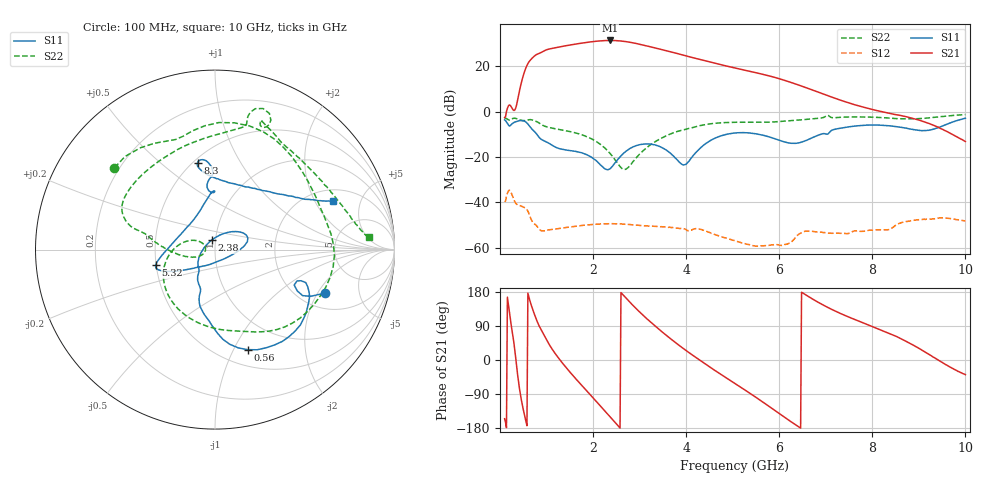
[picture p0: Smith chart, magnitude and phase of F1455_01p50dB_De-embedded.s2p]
! Integrated Device Technology
! Corporate Headquarters
! 6024 Silver Creek Valley Road
! San Jose, CA 95138  USA
! Phone:  1-408-284-8200
! Toll Free:  1-800-223-1366
! Webpage:  http://www.idt.com/
! Timing and RF Division
! 515 Groton Road, Suite 102
! Westford, MA 01886-6024
! Device:  F1455
! Description: 6-bit 0.5 dB Transmit Variable Gain Amplifier
! Frequency:  1400.0 -  2300.00 MHz
! Package:  6x6 mm Thin QFN Plastic Package: 28 pin
! State:  3
! Atten State:  1.5 dB
! Voltage:  +5.00 Volts
! Current:  214.186 mA
! Data:  The device was measured on a the F1455 evaluation board which has
!  individual transmission lines to the RF pins.  Data was collected
!  using a calibrated network analyzer.  The evaluation board was
!  de-embedded using a TRL calibration technique.
!  The reference plane is the edge of the package pin.
!  Pin  1 = CSb
!  Pin  2 = DATA
!  Pin  3 = CLK
!  Pin  4 = RSET
!  Pin  5 = GND
!  Pin  6 = RFIN  = Port 1
!  Pin  7 = GND
!  Pin  8 = NC
!  Pin  9 = NC
!  Pin 10 = NC
!  Pin 11 = NC
!  Pin 12 = NC
!  Pin 13 = NC
!  Pin 14 = /STBY
!  Pin 15 = GND
!  Pin 16 = RFOUT  = Port 2
!  Pin 17 = GND
!  Pin 18 = NC
!  Pin 19 = NC
!  Pin 20 = NC
!  Pin 21 = GND
!  Pin 22 = NC
!  Pin 23 = GND
!  Pin 24 = NC
!  Pin 25 = NC
!  Pin 26 = NC
!  Pin 27 = GND
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# GHz S dB R 50
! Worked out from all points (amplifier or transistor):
!   496 points, 100 MHz to 10 GHz, reference 50 ohm
!   highest |S21| = 31.4 dB at 2.36 GHz (marker M1)
!   |S21| within 3 dB of that: 1.242 GHz to 3.272 GHz (2.03 GHz wide, 89.9 % of centre)
!   unconditionally stable (mu >= 1): start of sweep to end of sweep
!   at 1.74 GHz: K = 4.55, MAG = 30.7 dB, |S12| = -50.3 dB
!   at 5.06 GHz: K = 23.08, MAG = 21.5 dB, |S12| = -57.1 dB
!   at 10 GHz: K = 74.51, MAG = -4.2 dB, |S12| = -48.3 dB
!   S11 on the Smith chart (normalised r, x): 100 MHz: 2.70, -2.31; 560 MHz: 0.67, -1.14; 2.38 GHz: 0.96, +0.10; 5.32 GHz: 0.50, -0.10; 8.3 GHz: 0.53, +0.67; 10 GHz: 2.59, +2.87
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0.1  -3.64 -21.6  -2.60 -154.9  -39.83 39.5  -2.83 140.8
0.4  -4.06 -38.1  7.21 -58.8  -41.27 -110.5  -3.44 50.6
0.56  -4.64 -72.0  19.46 -163.0  -42.82 -164.7  -3.92 16.5
0.7  -7.98 -94.7  23.77 134.7  -48.69 153.1  -3.72 -19.1
0.96  -12.99 -111.9  26.94 62.8  -52.59 125.8  -6.42 -72.2
1.14  -15.08 -123.1  28.00 25.2  -51.94 104.4  -7.36 -96.3
1.34  -16.63 -127.0  28.81 -7.7  -51.41 83.1  -8.13 -119.5
1.76  -18.18 -141.0  30.25 -67.5  -50.25 49.2  -10.21 -158.1
2.06  -21.49 -164.1  31.06 -107.9  -49.72 29.6  -13.08 177.3
2.36  -25.30 114.5  31.42 -149.2  -49.48 10.8  -18.31 155.1
2.38  -24.98 107.7  31.42 -152.0  -49.46 9.4  -18.79 154.1
2.62  -19.08 56.6  31.13 175.2  -49.60 -3.9  -25.10 166.2
2.9  -15.23 34.0  30.20 138.9  -50.06 -17.9  -21.02 -157.1
3.12  -14.28 22.5  29.19 112.9  -50.37 -27.1  -16.46 -163.8
3.4  -15.12 10.5  27.77 82.7  -50.75 -38.2  -12.49 -176.8
4.02  -22.79 -91.6  24.48 23.1  -52.47 -64.8  -7.64 166.7
5.06  -9.40 -161.1  19.22 -62.9  -57.09 -99.3  -4.70 148.8
5.32  -9.34 -165.4  18.02 -83.8  -58.61 -99.3  -4.68 139.9
6.7  -11.61 103.3  9.66 162.1  -52.80 -128.2  -3.20 78.3
8.3  -6.13 101.4  -0.49 73.1  -52.18 173.1  -2.75 64.0
8.36  -6.23 101.7  -0.77 70.1  -52.07 175.5  -2.83 62.5
10  -2.93 22.4  -13.19 -38.7  -48.32 88.7  -1.29 4.6
